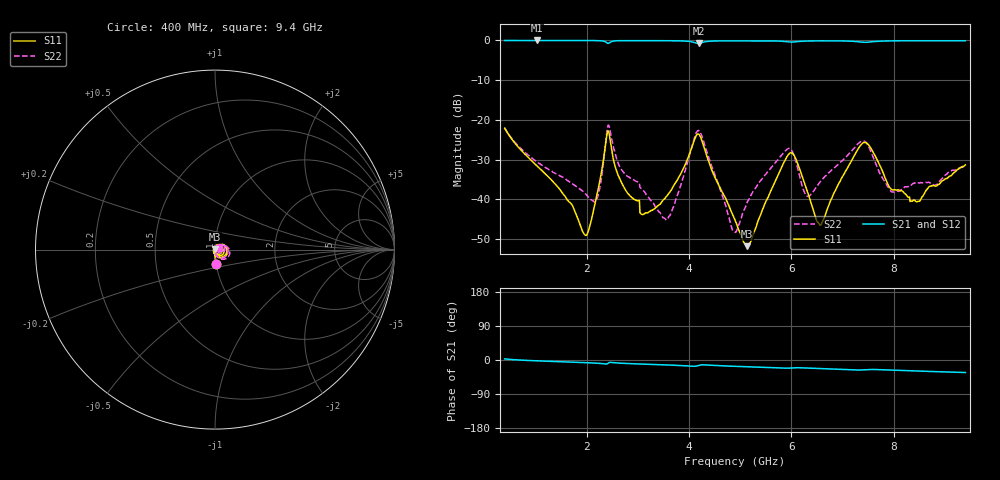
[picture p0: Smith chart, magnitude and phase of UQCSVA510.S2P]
!  Part Number  UQCSVA510  Mounting Orientation: Horizontal
!  Description: Ultra Low ESR Microwave capacitors
!  Application: Coupling, Bypass, Tuning, DC Block
!  Filters, Matching
# GHZ S DB R 50
! Freq  |S11|  S11 Ph  |S21|  S21 Ph  |S12|  S12 Ph  |S22|  S22 Ph
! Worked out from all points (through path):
!   801 points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, 400 MHz to 9.4 GHz, reference 50 ohm
!   highest |S21| = -0.03 dB at 1.03 GHz (marker M1); lowest = -0.8 dB at 4.191 GHz (marker M2)
!   group delay of S21, straight-line fit = 9.97 ps
!   lowest |S11| = -51.8 dB at 5.136 GHz (marker M3), VSWR 1.01, Z = 49.8 + j0.146 ohm
!   |S11| at or under -10 dB: start of sweep to end of sweep
!   |S22| runs from -48.4 to -21.3 dB; largest |S21 - S12| = 0.0014
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0.4  -22.13 -86.4  -0.04 3.0  -0.05 3.0  -22.00 -84.8
1.03  -31.59 -94.7  -0.03 -2.2  -0.03 -2.2  -30.61 -83.8
1.694  -41.04 -114.9  -0.04 -5.6  -0.05 -5.6  -35.83 -70.4
1.908  -47.60 -154.2  -0.05 -6.6  -0.05 -6.6  -37.75 -59.0
2.02  -48.56 151.9  -0.05 -7.2  -0.06 -7.2  -39.21 -48.2
2.2  -39.12 88.9  -0.08 -8.4  -0.08 -8.4  -39.86 -0.5
2.425  -22.82 -18.7  -0.77 -8.0  -0.78 -8.0  -21.33 -16.3
2.65  -34.92 -108.4  -0.08 -8.3  -0.08 -8.3  -31.87 -72.7
3.089  -43.87 178.8  -0.07 -10.8  -0.07 -10.8  -37.51 -63.7
3.404  -41.56 126.9  -0.09 -12.3  -0.09 -12.2  -43.04 -40.1
3.629  -38.16 103.6  -0.10 -13.4  -0.11 -13.4  -44.11 18.1
4.191  -23.61 -20.4  -0.77 -14.3  -0.77 -14.3  -22.70 -18.6
4.9  -45.23 -147.6  -0.12 -16.7  -0.12 -16.7  -48.28 172.6
5.136  -51.82 145.1  -0.12 -17.8  -0.12 -17.8  -40.83 107.4
5.969  -28.43 -14.1  -0.41 -21.3  -0.42 -21.3  -27.27 23.2
6.261  -36.12 -77.0  -0.19 -21.0  -0.19 -21.0  -38.41 3.8
6.408  -41.83 -70.9  -0.15 -21.8  -0.15 -21.8  -38.25 39.5
6.599  -45.84 -9.1  -0.13 -22.8  -0.13 -22.8  -35.10 53.7
7.42  -25.72 -19.5  -0.49 -25.9  -0.49 -25.9  -25.34 -0.9
7.904  -36.72 -58.6  -0.15 -26.5  -0.15 -26.5  -37.17 -23.4
8.478  -40.56 -5.2  -0.09 -29.2  -0.09 -29.1  -35.86 10.0
9.4  -31.36 23.9  -0.11 -33.0  -0.11 -33.0  -31.61 24.6
